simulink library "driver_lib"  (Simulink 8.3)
settings: Solver=ode45  StartTime=0.0  StopTime=10.0  RelTol=1e-3
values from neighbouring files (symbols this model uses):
  driver = class_REVS_driver    [driver_param.m]    (also in REVS_run_preproc.m)
undefined symbols (not defined in the file or in its folder): convert, drive_cycle, REVS
libraries: simulink x14, general_lib x13

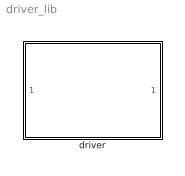
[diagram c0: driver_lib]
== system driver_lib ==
  driver : Subsystem  VariantControl=variants_driver_MT

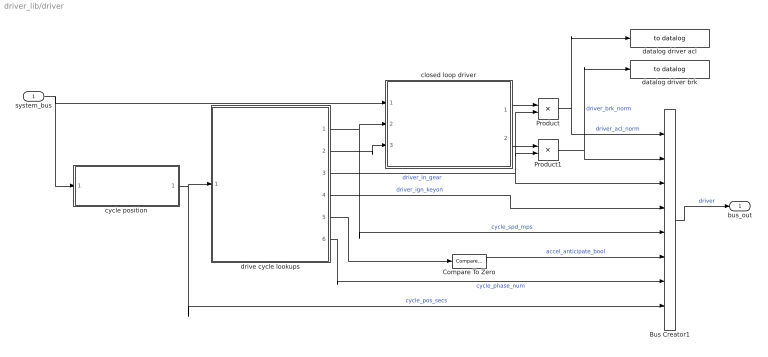
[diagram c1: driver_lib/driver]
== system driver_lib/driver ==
  system_bus : Inport
  Bus Creator1 : BusCreator  Inputs=8
  Compare To Zero : simulink/Logic and Bit Operations/Compare To Zero  relop=>  OutDataTypeStr=boolean
  Product : Product
  Product1 : Product
  closed loop driver : Subsystem
  cycle position : Subsystem
  datalog driver acl : general_lib/to datalog  VarName=driver__accel_norm  WorkspaceName=datalog__driver__accel_norm  VerboseLevel=1  VerboseSignal=REVS.verbose
  datalog driver brk : general_lib/to datalog  VarName=driver__brake_norm  WorkspaceName=datalog__driver__brake_norm  VerboseLevel=1  VerboseSignal=REVS.verbose
  drive cycle lookups : Subsystem
  bus_out : Outport
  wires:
  Compare To Zero/1 -> Bus Creator1/6  "accel_anticipate_bool"
  drive cycle lookups/5(anticipate_veh_spd_des_mps) -> Compare To Zero/1
  cycle position/1(cycle_position_secs) -> drive cycle lookups/1(cycle_position_secs), Bus Creator1/8  "cycle_pos_secs"
  drive cycle lookups/3(driver_in_gear) -> Bus Creator1/3, Product1/2, Product/2  "driver_in_gear"
  Product1/1 -> Bus Creator1/2, datalog driver brk/1  "driver_brk_norm"
  Product/1 -> Bus Creator1/1, datalog driver acl/1  "driver_acl_norm"
  drive cycle lookups/4(driver_key_pos) -> Bus Creator1/4  "driver_ign_keyon"
  closed loop driver/2(brk_pedal_norm) -> Product1/1
  closed loop driver/1(acl_pedal_norm) -> Product/1
  Bus Creator1/1 -> bus_out/1  "driver"
  system_bus/1 -> closed loop driver/1(system_bus), cycle position/1(system_bus)
  drive cycle lookups/2(future_veh_spd_des_mps) -> closed loop driver/3(future_veh_spd_des_mps)
  drive cycle lookups/1(veh_spd_des_mps) -> Bus Creator1/5, closed loop driver/2(veh_spd_des_mps)  "cycle_spd_mps"
  drive cycle lookups/6(cycle_phase) -> Bus Creator1/7  "cycle_phase_num"

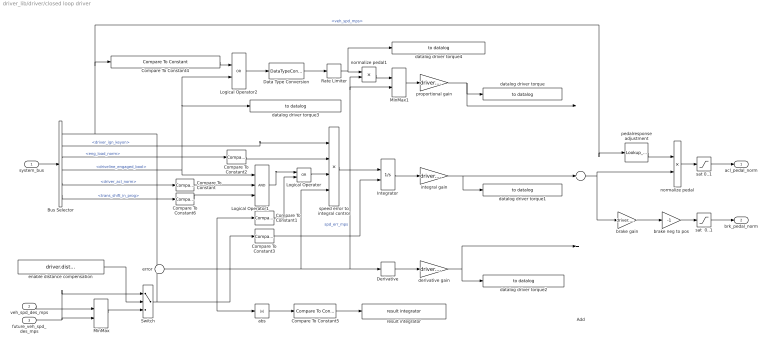
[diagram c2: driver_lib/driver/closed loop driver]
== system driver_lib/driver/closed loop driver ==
  system_bus : Inport
  veh_spd_des_mps : Inport  Port=2
  future_veh_spd_des_mps : Inport  Port=3
  Add : Sum  Inputs=+++
  Bus Selector : BusSelector  OutputSignals=vehicle.veh_spd_mps,driver.driver_ign_keyon,powertrain.engine.eng_load_norm,powertrain.trans.ctrl.core_ctl.driveline_engaged_bool,driver.driver_acl_norm,powertrain.trans.ctrl.core_ctl.trans_shift_in_prog
  Compare To Constant : simulink/Logic and Bit Operations/Compare To Constant  relop=<  const=1  OutDataTypeStr=boolean  ZeroCross=off
  Compare To Constant1 : simulink/Logic and Bit Operations/Compare To Constant  relop=<  const=0  OutDataTypeStr=boolean  ZeroCross=off
  Compare To Constant2 : simulink/Logic and Bit Operations/Compare To Constant  relop=<  const=0.99  OutDataTypeStr=boolean  ZeroCross=off
  Compare To Constant3 : simulink/Logic and Bit Operations/Compare To Constant  relop=<=  const=0  OutDataTypeStr=boolean  ZeroCross=off
  Compare To Constant4 : simulink/Logic and Bit Operations/Compare To Constant  relop=<  const=driver.proportional_fade_in_min_speed_mps  OutDataTypeStr=boolean  ZeroCross=off
  Compare To Constant5 : simulink/Logic and Bit Operations/Compare To Constant  relop=>  const=2*convert.mph2mps  OutDataTypeStr=boolean  ZeroCross=off
  Compare To Constant6 : simulink/Logic and Bit Operations/Compare To Constant  relop===  const=0  OutDataTypeStr=boolean  ZeroCross=off
  Data Type Conversion : DataTypeConversion
  Derivative : Derivative
  Integrator : Integrator  ExternalReset=level  LimitOutput=on  LowerSaturationLimit=0  ZeroCross=off
  Logical Operator : Logic  Operator=OR  AllPortsSameDT=off  OutDataTypeStr=boolean
  Logical Operator1 : Logic  Inputs=3  AllPortsSameDT=off  OutDataTypeStr=boolean
  Logical Operator2 : Logic  Operator=OR  AllPortsSameDT=off  OutDataTypeStr=boolean
  MinMax : MinMax  Function=max  Inputs=2  ZeroCross=off
  MinMax1 : MinMax  Inputs=2  ZeroCross=off
  Rate Limiter : RateLimiter  RisingSlewLimit=1/driver.proportional_fade_in_secs  FallingSlewLimit=-inf  LinearizeAsGain=off
  Switch : Switch  Criteria=u2 ~= 0  ZeroCross=off
  abs : Abs
  brake gain : Gain  Gain=driver.brake_gain_norm
  brake neg to pos : Gain  Gain=-1
  datalog driver torque : general_lib/to datalog  VarName=driver.p_pedal_unscaled  WorkspaceName=datalog__driver__p_pedal_unscaled  VerboseLevel=3  VerboseSignal=REVS.verbose
  datalog driver torque1 : general_lib/to datalog  VarName=driver.i_pedal_unscaled  WorkspaceName=datalog__driver__i_pedal_unscaled  VerboseLevel=3  VerboseSignal=REVS.verbose
  datalog driver torque2 : general_lib/to datalog  VarName=driver.d_pedal_unscaled  WorkspaceName=datalog__driver__d_pedal_unscaled  VerboseLevel=3  VerboseSignal=REVS.verbose
  datalog driver torque3 : general_lib/to datalog  VarName=driver.driveline_enagaged_bool  WorkspaceName=datalog__driver__driveline_enagaged_bool  VerboseLevel=3  VerboseSignal=REVS.verbose
  datalog driver torque4 : general_lib/to datalog  VarName=driver.driveline_enagaged_norm  WorkspaceName=datalog__driver__driveline_enagaged_norm  VerboseLevel=3  VerboseSignal=REVS.verbose
  derivative gain : Gain  Gain=driver.Kd
  enable distance compensation : Constant  Value=driver.distance_compensate_enable
  error : Sum  Inputs=-+
  integral gain : Gain  Gain=driver.Ki/100
  normalize pedal : Product  Inputs=**
  normalize pedal1 : Product  Inputs=**
  pedalresponse adjustment : Lookup_n-D  NumberOfTableDimensions=1  BreakpointsForDimension1=driver.accel_pedal_response_speed_mps  IndexSearchMethod=Linear search  BeginIndexSearchUsingPreviousIndexResult=on  Table=driver.accel_pedal_response_norm  ExtrapMethod=Clip  UseLastTableValue=on  RndMeth=Simplest
  proportional gain : Gain  Description=1.3 factor converts REVS1 Kp to REVS2 Kp, more or less  RequirementInfo={} %GIDa_c10416ae_7039_4e6e_8729_c37e926f399b  Gain=driver.Kp * 1.3
  result integrator : general_lib/result integrator  ResultSignalName=driver_error_time_secs  ResultBaseName=''
  sat  0..1 : Saturate  UpperLimit=1  LowerLimit=0  ZeroCross=off
  sat 0..1 : Saturate  UpperLimit=1  LowerLimit=0  ZeroCross=off
  speed error to integral control : Product  Inputs=4
  acl_pedal_norm : Outport
  brk_pedal_norm : Outport  Port=2
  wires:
  Bus Selector/6 -> Compare To Constant6/1  "<trans_shift_in_prog>"
  Compare To Constant6/1 -> Logical Operator1/3
  Logical Operator2/1 -> Data Type Conversion/1
  normalize pedal1/1 -> MinMax1/1
  proportional gain/1 -> Add/1, datalog driver torque/1
  brake gain/1 -> brake neg to pos/1
  sat  0..1/1 -> brk_pedal_norm/1
  sat 0..1/1 -> acl_pedal_norm/1
  Add/1 -> normalize pedal/2, brake gain/1
  normalize pedal/1 -> sat 0..1/1
  pedalresponse adjustment/1 -> normalize pedal/1
  Bus Selector/2 -> speed error to integral control/1  "<driver_ign_keyon>"
  MinMax/1 -> Switch/3
  enable distance compensation/1 -> Switch/2
  future_veh_spd_des_mps/1 -> MinMax/2, Switch/1
  Bus Selector/1 -> error/1, Compare To Constant4/1, pedalresponse adjustment/1  "<veh_spd_mps>"
  Bus Selector/4 -> Logical Operator1/1, datalog driver torque3/1, Logical Operator2/2  "<driveline_engaged_bool>"
  derivative gain/1 -> datalog driver torque2/1, Add/3
  integral gain/1 -> datalog driver torque1/1, Add/2
  error/1 -> Compare To Constant1/1, abs/1, speed error to integral control/4, Derivative/1, normalize pedal1/2, MinMax1/2  "spd_err_mps"
  speed error to integral control/1 -> Integrator/1
  system_bus/1 -> Bus Selector/1
  veh_spd_des_mps/1 -> MinMax/1
  Derivative/1 -> derivative gain/1
  Integrator/1 -> integral gain/1
  Bus Selector/5 -> Compare To Constant/1  "<driver_acl_norm>"
  Compare To Constant/1 -> Logical Operator1/2
  Compare To Constant1/1 -> Logical Operator/2
  Logical Operator/1 -> speed error to integral control/3
  Bus Selector/3 -> Compare To Constant2/1  "<eng_load_norm>"
  Compare To Constant2/1 -> speed error to integral control/2
  Switch/1 -> Compare To Constant3/1, error/2
  Compare To Constant3/1 -> Integrator/2
  Logical Operator1/1 -> Logical Operator/1
  Compare To Constant4/1 -> Logical Operator2/1
  Rate Limiter/1 -> datalog driver torque4/1, normalize pedal1/1
  MinMax1/1 -> proportional gain/1
  Data Type Conversion/1 -> Rate Limiter/1
  Compare To Constant5/1 -> result integrator/1
  abs/1 -> Compare To Constant5/1
  brake neg to pos/1 -> sat  0..1/1

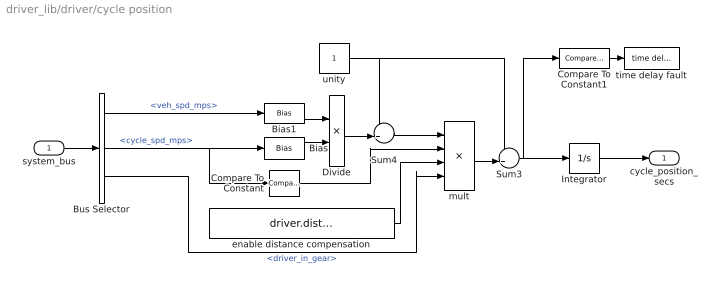
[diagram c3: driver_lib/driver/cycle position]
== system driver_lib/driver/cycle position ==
  system_bus : Inport
  Bias : Bias  Bias=eps
  Bias1 : Bias  Bias=eps
  Bus Selector : BusSelector  OutputSignals=vehicle.veh_spd_mps,driver.cycle_spd_mps,driver.driver_in_gear
  Compare To Constant : simulink/Logic and Bit Operations/Compare To Constant  relop=>=  const=1.0  OutDataTypeStr=boolean  ZeroCross=off
  Compare To Constant1 : simulink/Logic and Bit Operations/Compare To Constant  relop=<=  const=1e-9  OutDataTypeStr=boolean
  Divide : Product  Inputs=*/
  Integrator : Integrator  InitialCondition=REVS.sim_start_time_secs
  Sum3 : Sum  Inputs=++|
  Sum4 : Sum  Inputs=-+|
  enable distance compensation : Constant  Value=driver.distance_compensate_enable
  mult : Product  Inputs=4
  time delay fault : general_lib/time delay fault  DelayTimeSecs=10  ErrorCallBack=error('Klaatu Berada Nicto')
  unity : Constant
  cycle_position_secs : Outport
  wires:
  Bus Selector/3 -> mult/4  "<driver_in_gear>"
  Compare To Constant1/1 -> time delay fault/1
  mult/1 -> Sum3/2
  enable distance compensation/1 -> mult/3
  Bus Selector/2 -> Bias/1, Compare To Constant/1  "<cycle_spd_mps>"
  system_bus/1 -> Bus Selector/1
  Bus Selector/1 -> Bias1/1  "<veh_spd_mps>"
  Sum4/1 -> mult/1
  Compare To Constant/1 -> mult/2
  unity/1 -> Sum3/1, Sum4/1
  Divide/1 -> Sum4/2
  Sum3/1 -> Integrator/1, Compare To Constant1/1
  Bias/1 -> Divide/2
  Bias1/1 -> Divide/1
  Integrator/1 -> cycle_position_secs/1

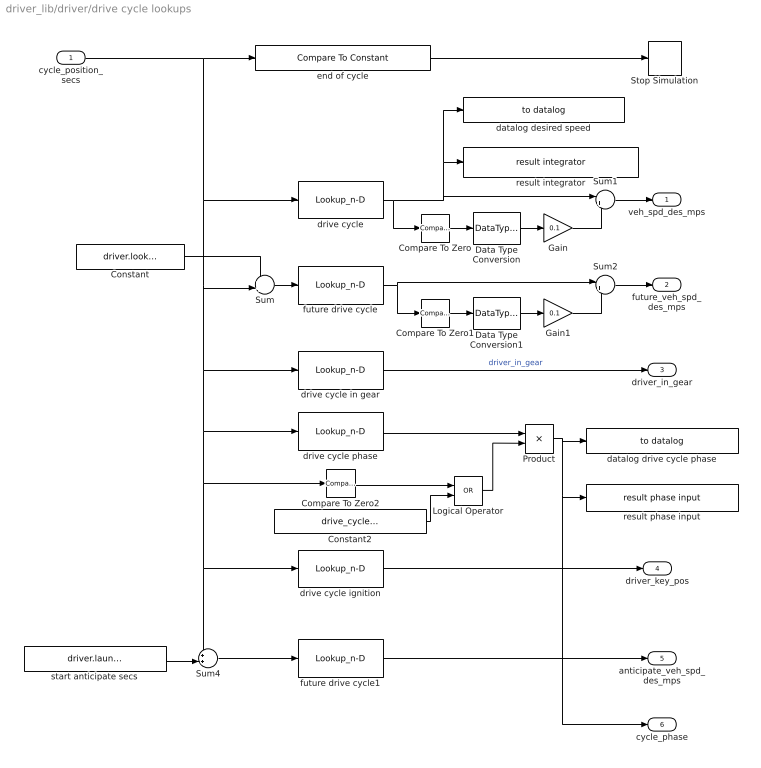
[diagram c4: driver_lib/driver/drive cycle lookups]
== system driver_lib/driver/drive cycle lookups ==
  cycle_position_secs : Inport
  Compare To Zero : simulink/Logic and Bit Operations/Compare To Zero  relop=<=  OutDataTypeStr=uint8  ZeroCross=off
  Compare To Zero1 : simulink/Logic and Bit Operations/Compare To Zero  relop=<=  OutDataTypeStr=uint8  ZeroCross=off
  Compare To Zero2 : simulink/Logic and Bit Operations/Compare To Zero  relop=>=  OutDataTypeStr=boolean
  Constant : Constant  Value=driver.lookahead_secs
  Constant2 : Constant  Value=drive_cycle.sample_start_enable
  Data Type Conversion : DataTypeConversion
  Data Type Conversion1 : DataTypeConversion
  Gain : Gain  Gain=0.1
  Gain1 : Gain  Gain=0.1
  Logical Operator : Logic  Operator=OR  AllPortsSameDT=off  OutDataTypeStr=boolean
  Product : Product
  Stop Simulation : Stop
  Sum : Sum  Inputs=++|
  Sum1 : Sum  Inputs=|+-
  Sum2 : Sum  Inputs=|+-
  Sum4 : Sum  Inputs=++|
  datalog desired speed : general_lib/to datalog  VarName=drive_cycle_speed_mps  WorkspaceName=datalog__drive_cycle_speed_mps  VerboseLevel=0  VerboseSignal=REVS.verbose
  datalog drive cycle phase : general_lib/to datalog  VarName=drive_cycle_phase  WorkspaceName=datalog__drive_cycle_phase  VerboseLevel=0  VerboseSignal=REVS.verbose
  drive cycle : Lookup_n-D  NumberOfTableDimensions=1  BreakpointsForDimension1=drive_cycle.cycle_time  IndexSearchMethod=Linear search  BeginIndexSearchUsingPreviousIndexResult=on  Table=drive_cycle.cycle_speed_mps  ExtrapMethod=Clip  UseLastTableValue=on  RndMeth=Simplest  MaximumIndicesForEachDimension=1e5
  drive cycle ignition : Lookup_n-D  NumberOfTableDimensions=1  BreakpointsForDimension1=drive_cycle.ignition_time  IndexSearchMethod=Linear search  BeginIndexSearchUsingPreviousIndexResult=on  Table=drive_cycle.ignition  InterpMethod=Flat  ExtrapMethod=Clip  UseLastTableValue=on  RndMeth=Simplest  MaximumIndicesForEachDimension=1e5
  drive cycle in gear : Lookup_n-D  NumberOfTableDimensions=1  BreakpointsForDimension1=drive_cycle.in_gear_time  IndexSearchMethod=Linear search  BeginIndexSearchUsingPreviousIndexResult=on  Table=drive_cycle.in_gear  InterpMethod=Flat  ExtrapMethod=Clip  UseLastTableValue=on  RndMeth=Simplest  MaximumIndicesForEachDimension=1e5
  drive cycle phase : Lookup_n-D  NumberOfTableDimensions=1  BreakpointsForDimension1=drive_cycle.phase_time  IndexSearchMethod=Linear search  BeginIndexSearchUsingPreviousIndexResult=on  Table=drive_cycle.phase  InterpMethod=Flat  ExtrapMethod=Clip  UseLastTableValue=on  RndMeth=Simplest  MaximumIndicesForEachDimension=1e5
  end of cycle : simulink/Logic and Bit Operations/Compare To Constant  relop=>=  const=drive_cycle.cycle_time(end)  OutDataTypeStr=boolean
  future drive cycle : Lookup_n-D  NumberOfTableDimensions=1  BreakpointsForDimension1=drive_cycle.cycle_time  IndexSearchMethod=Linear search  BeginIndexSearchUsingPreviousIndexResult=on  Table=drive_cycle.cycle_speed_mps  ExtrapMethod=Clip  UseLastTableValue=on  RndMeth=Simplest  MaximumIndicesForEachDimension=1e5
  future drive cycle1 : Lookup_n-D  NumberOfTableDimensions=1  BreakpointsForDimension1=drive_cycle.cycle_time  IndexSearchMethod=Linear search  BeginIndexSearchUsingPreviousIndexResult=on  Table=drive_cycle.cycle_speed_mps  ExtrapMethod=Clip  UseLastTableValue=on  RndMeth=Simplest  MaximumIndicesForEachDimension=1e5
  result integrator : general_lib/result integrator  ResultSignalName=drive_cycle_distance_m  ResultBaseName=''
  result phase input : general_lib/result phase input  NumPhases=max(drive_cycle.phase)  ResultTimeOutput=time_secs
  start anticipate secs : Constant  Value=driver.launch_anticipate_secs
  veh_spd_des_mps : Outport
  future_veh_spd_des_mps : Outport  Port=2
  driver_in_gear : Outport  Port=3
  driver_key_pos : Outport  Port=4
  anticipate_veh_spd_des_mps : Outport  Port=5
  cycle_phase : Outport  Port=6
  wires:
  future drive cycle1/1 -> anticipate_veh_spd_des_mps/1
  cycle_position_secs/1 -> drive cycle in gear/1, drive cycle phase/1, drive cycle ignition/1, Sum4/1, Compare To Zero2/1, Sum/2, drive cycle/1, end of cycle/1
  start anticipate secs/1 -> Sum4/2
  Sum4/1 -> future drive cycle1/1
  drive cycle ignition/1 -> driver_key_pos/1
  Constant2/1 -> Logical Operator/2
  Logical Operator/1 -> Product/2
  Compare To Zero2/1 -> Logical Operator/1
  Product/1 -> cycle_phase/1, result phase input/1, datalog drive cycle phase/1
  drive cycle phase/1 -> Product/1
  end of cycle/1 -> Stop Simulation/1
  drive cycle in gear/1 -> driver_in_gear/1  "driver_in_gear"
  Constant/1 -> Sum/1
  drive cycle/1 -> Compare To Zero/1, Sum1/1, result integrator/1, datalog desired speed/1
  future drive cycle/1 -> Compare To Zero1/1, Sum2/1
  Sum/1 -> future drive cycle/1
  Sum1/1 -> veh_spd_des_mps/1
  Sum2/1 -> future_veh_spd_des_mps/1
  Compare To Zero/1 -> Data Type Conversion/1
  Compare To Zero1/1 -> Data Type Conversion1/1
  Gain/1 -> Sum1/2
  Gain1/1 -> Sum2/2
  Data Type Conversion/1 -> Gain/1
  Data Type Conversion1/1 -> Gain1/1
